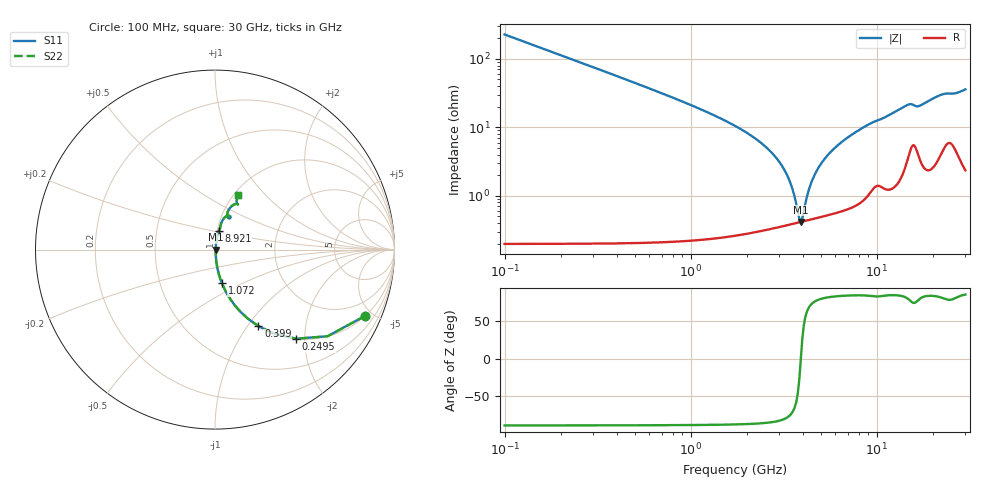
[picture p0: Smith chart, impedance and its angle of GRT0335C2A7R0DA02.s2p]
!Murata Part Number: GRT0335C2A7R0DA02
!These Parameters are Measured in Series Mode Connection
!Data Generated on Jun 19, 2026
!  o--ll--o
!Port1  Port2
!  o------o
!Operation Temp=25[degC], DC Bias Voltage=0[V]
!Freq. Start=100[MHz] Stop=30[GHz] 401[Steps]
# Hz S RI R 50
!Freq.(Hz) S11(Real) S11(Imag) S21(Real) S21(Imag) S12(Real) S12(Imag) S22(Real) S22(Imag)
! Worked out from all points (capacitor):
!   401 points, 100 MHz to 30 GHz, reference 50 ohm
!   read as one part in series: C = 7 pF near 249.5 MHz
!   lowest |Z| = 414 mohm at 3.912 GHz (marker M1)
!   series resonance near 3.913 GHz, so ESL is about 240 pH
!   S11 on the Smith chart (normalised r, x): 100 MHz: 1.00, -4.54; 249.5 MHz: 1.00, -1.81; 399 MHz: 1.00, -1.13; 1.072 GHz: 1.00, -0.39; 8.921 GHz: 1.02, +0.21; 30 GHz: 1.05, +0.72
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1e8  0.8375 -0.3685  0.1625 0.3685  0.1625 0.3685  0.8375 -0.3685
2.495e8  0.4517 -0.4966  0.5483 0.4966  0.5483 0.4966  0.4517 -0.4966
3.99e8  0.242 -0.4265  0.758 0.4265  0.758 0.4265  0.242 -0.4265
6.2325e8  0.1135 -0.3143  0.8865 0.3143  0.8865 0.3143  0.1135 -0.3143
1.07175e9  0.0389 -0.1878  0.9611 0.1878  0.9611 0.1878  0.0389 -0.1878
2.492e9  0.00598 -0.0534  0.994 0.0534  0.994 0.0534  0.00598 -0.0534
3.01525e9  0.0044 -0.0301  0.9956 0.0301  0.9956 0.0301  0.0044 -0.0301
3.389e9  0.00403 -0.0165  0.996 0.0165  0.996 0.0165  0.00403 -0.0165
3.76275e9  0.00404 -0.00446  0.996 0.00446  0.996 0.00446  0.00404 -0.00446
3.91225e9  0.00413 -1.93e-05  0.9959 1.93e-05  0.9959 1.93e-05  0.00413 -1.93e-05
4.06175e9  0.00425 0.00425  0.9958 -0.00425  0.9958 -0.00425  0.00425 0.00425
4.286e9  0.00449 0.0104  0.9955 -0.0104  0.9955 -0.0104  0.00449 0.0104
4.51025e9  0.0048 0.0162  0.9952 -0.0162  0.9952 -0.0162  0.0048 0.0162
5.10825e9  0.00587 0.0306  0.9941 -0.0306  0.9941 -0.0306  0.00587 0.0306
6.5285e9  0.00962 0.0606  0.9904 -0.0606  0.9904 -0.0606  0.00962 0.0606
8.9205e9  0.0208 0.1042  0.9792 -0.1042  0.9792 -0.1042  0.0208 0.1042
1.01165e10  0.0286 0.12  0.9714 -0.12  0.9714 -0.12  0.0286 0.12
1.505e10  0.0797 0.1882  0.9203 -0.1882  0.9203 -0.1882  0.0797 0.1882
1.66945e10  0.0726 0.1774  0.9274 -0.1774  0.9274 -0.1774  0.0726 0.1774
2.005825e10  0.0846 0.2335  0.9154 -0.2335  0.9154 -0.2335  0.0846 0.2335
2.50665e10  0.1275 0.2519  0.8725 -0.2519  0.8725 -0.2519  0.1275 0.2519
3e10  0.1293 0.3042  0.8707 -0.3042  0.8707 -0.3042  0.1293 0.3042
